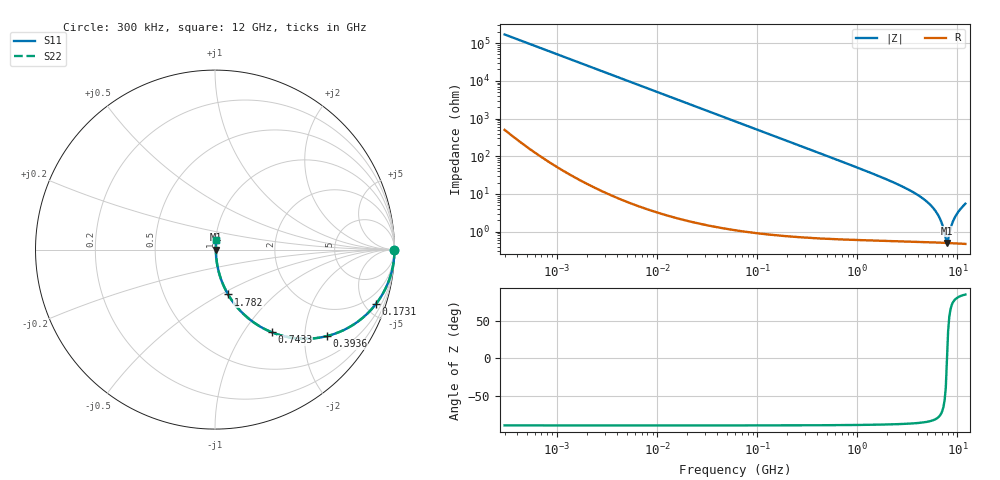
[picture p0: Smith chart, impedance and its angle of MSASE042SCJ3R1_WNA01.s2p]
! MSASE042SCJ3R1_WNA01  S-PARAMETER MODEL  ( General Type )
! Model Generated by TAIYO YUDEN Corporation (http://www.ty-top.com)
! Version 1.0
! TAIYO YUDEN Control No. 120810
! Copyright(c) 2012 TAIYO YUDEN CO.,LTD. All Rights Reserved.
! Product Description (link to TY-COMPAS)
! https://ds.yuden.co.jp/TYCOMPAS/or/detail?pn=MSASE042SCJ3R1BWNA01&u=M
! Products Name : Multilayer Ceramic Capacitors
! Characteristics :
!  Capacitance : 3.1 pF , Rated Voltage : 16V , TCC : CJ / C0J
!  Case Size : 0.4 x 0.2 / 0.016 x 0.008 [mm/inch] , Thickness : 0.2 / 0.008 [mm/inch]
!  (Conditions: Temperature = 25 degC , DC Bias Current/Voltage = 0A / 0V)
! External Node Assignments :
!  1  o---| |---o  2
! GND o---------o GND
! Frequency Range : 0.3MHz  -  12000MHz  [ 401 STEP ]
# MHz S RI R 50
! Freq[MHz].  S11 Real  S11 Imag  S21 Real  S21 Imag  S12 Real  S12 Imag  S22 Real  S22 Imag
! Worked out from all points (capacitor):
!   401 points, 300 kHz to 12 GHz, reference 50 ohm
!   read as one part in series: C = 3.13 pF near 316.3 kHz
!   lowest |Z| = 502 mohm at 7.854 GHz (marker M1)
!   series resonance near 7.853 GHz, so ESL is about 130 pH
!   S11 on the Smith chart (normalised r, x): 300 kHz: open; 173.1 MHz: 1.02, -5.88; 393.6 MHz: 1.01, -2.57; 743.3 MHz: 1.01, -1.36; 1.782 GHz: 1.01, -0.54; 12 GHz: 1.01, +0.11
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0.3  1 -0.00059  2.09e-06 0.00059  2.09e-06 0.00059  1 -0.00059
1.769972  1 -0.00348  1.47e-05 0.00348  1.47e-05 0.00348  1 -0.00348
10.44266  0.9996 -0.0205  0.000434 0.0205  0.000434 0.0205  0.9996 -0.0205
60  0.9861 -0.1163  0.0139 0.1163  0.0139 0.1163  0.9861 -0.1163
173.124  0.8955 -0.3046  0.1045 0.3046  0.1045 0.3046  0.8955 -0.3046
353.9943  0.6722 -0.467  0.3278 0.467  0.3278 0.467  0.6722 -0.467
393.5654  0.6231 -0.482  0.3769 0.482  0.3769 0.482  0.6231 -0.482
743.2595  0.3168 -0.4607  0.6832 0.4607  0.6832 0.4607  0.3168 -0.4607
1135.593  0.1648 -0.3643  0.8352 0.3643  0.8352 0.3643  0.1648 -0.3643
1781.601  0.073 -0.2498  0.927 0.2498  0.927 0.2498  0.073 -0.2498
2088.533  0.0537 -0.2132  0.9463 0.2132  0.9463 0.2132  0.0537 -0.2132
3642.919  0.0171 -0.1075  0.9829 0.1075  0.9829 0.1075  0.0171 -0.1075
5278.635  0.00801 -0.0526  0.992 0.0526  0.992 0.0526  0.00801 -0.0526
6524.734  0.00571 -0.0244  0.9943 0.0244  0.9943 0.0244  0.00571 -0.0244
7064.448  0.00526 -0.0142  0.9947 0.0142  0.9947 0.0142  0.00526 -0.0142
7448.838  0.00509 -0.0074  0.9949 0.0074  0.9949 0.0074  0.00509 -0.0074
7854.144  0.005 2.63e-05  0.995 -2.63e-05  0.995 -2.63e-05  0.005 2.63e-05
8281.503  0.00502 0.00708  0.995 -0.00708  0.995 -0.00708  0.00502 0.00708
8966.534  0.00522 0.0173  0.9948 -0.0173  0.9948 -0.0173  0.00522 0.0173
9454.42  0.00545 0.0238  0.9946 -0.0238  0.9946 -0.0238  0.00545 0.0238
10793.46  0.0064 0.04  0.9936 -0.04  0.9936 -0.04  0.0064 0.04
12000  0.0077 0.0544  0.9923 -0.0544  0.9923 -0.0544  0.0077 0.0544
